(* Logix 5000 AddOnInstructionDefinition export AMCI_MA_SV_Circular_Follower; software revision 31.02 *)

TYPE AMCI_Motion_Axis_Input_Data :
STRUCT
   Moving_CW : BOOL;
   Moving_CCW : BOOL;
   In_Hold_State : BOOL;
   Stopped : BOOL;
   At_Home : BOOL;
   Accelerating : BOOL;
   Decelerating : BOOL;
   Move_Complete : BOOL;
   Status_Word_0_Bit_8 : BOOL;
   Status_Word_0_Bit_9 : BOOL;
   Position_Invalid : BOOL;
   Input_Error : BOOL;
   Command_Error : BOOL;
   Configuration_Error : BOOL;
   Module_OK : BOOL;
   Mode_Flag : BOOL;
   IN1_Active : BOOL;
   IN2_Active : BOOL;
   IN3_Active : BOOL;
   IN4_Active : BOOL;
   Status_Word_1_Bit_4 : BOOL;
   Status_Word_1_Bit_5 : BOOL;
   Connection_Was_Lost : BOOL;
   Driver_Fault : BOOL;
   Status_Word_1_Bit_8 : BOOL;
   Invalid_Jog_Change : BOOL;
   Status_Word_1_Bit_10 : BOOL;
   Heartbeat_Bit : BOOL;
   Status_Word_1_Bit_12 : BOOL;
   Status_Word_1_Bit_13 : BOOL;
   Stall_Detected : BOOL;
   Drive_Is_Enabled : BOOL;
   Motor_Position : DINT;
   Encoder_Position : DINT;
   Trapped_Encoder_Position : DINT;
   Input_Word_8 : INT;
   Input_Word_9 : INT;
END_STRUCT
END_TYPE

TYPE AMCI_Motion_Axis_Output_Data :
STRUCT
   Control_Word_0 : INT;
   Control_Word_1 : INT;
   Position_or_Distance : DINT;
   Programmed_Speed : DINT;
   Acceleration : INT;
   Deceleration : INT;
   Output_Word_8 : INT;
   Output_Word_9 : INT;
END_STRUCT
END_TYPE

ADD_ON_INSTRUCTION AMCI_MA_SV_Circular_Follower   (* revision 1.1, vendor AMCI, ExecuteEnableInFalse *)
// Only for SVXXXE2 motion devices.
// Revision note:
// Version 1.1:  Corrected mistake in the text on the Help Tab.   Also limited the velocity to +/-1,048,575 steps / sec.
// Help:
// MOTION AXIS SV CIRCULAR FOLLOWER
// These AOIs will only work with the SV motion devices.  The SMD and SD  motion devices have their own follower AOIs.
// AXIS INPUT DATA:  Input data from AMCI motion device.   Uses the AMCI_Motion_Axis_Input_Data User Defined Data Type.
// AXIS OUTPUT DATA; Output data from the AOI to the AMCI motion device.   Uses the AMCI_Motion_Axis_Output_Data User Defined Data Type.
// FOLLOWER POSITION: REAL DATA TYPE position directly from the motion axis.
// FOLLOWER VELOCITY: REAL DATA TYPE velocity directly from the motion axis.
// FOLLOWER ACCELERATION: REAL DATA TYPE acceleration directly from the motion axis.
// RAMP ACCELERATION: An actual value or INT value used to transition from no motion to motion.   Once
//                                          motion is occurring, the follower acceleration will be used.  Range of 0 to 15,999.
// DECELERATION: An actual value or INT value used to transition from motion to no motion.   Range of 0 to
//                              15,999.
// CONVERSION CONSTANT: Converts revolutions and revolutions / sec  from the motion axis to the step and
//                                               steps / sec used by the motion axis.
// POSITION UNWIND: Must be set to the Unwind Value of the motion axis and defines the point at which the
//                                    position data will transition from its maximum to its minimum value.    The Position
//                                    Unwind Value MUST BE IN THE RANGE OF 21 TO 65535.
// EN (Enable) Set when rung is true, Reset when rung is false
// DN (Done) Set when command is sent to the motion device.  Reset when the rung is false.
// ER (Error) Set when a command or input error failed to clear.  Reset when the rung is false.
// IP (In Process) Set when motion is occurring.   Reset when the rung goes false.
VAR_IN_OUT
   Axis_Input_Data : AMCI_Motion_Axis_Input_Data; {required}
   Axis_Output_Data : AMCI_Motion_Axis_Output_Data; {required}
END_VAR
VAR_INPUT
   Follower_Position : REAL; {required}
   Follower_Velocity : REAL; {required}
   Follower_Acceleration : REAL; {required}
   Ramp_Acceleration : INT; {required}
   Deceleration : INT; {required}
   Conversion_Constant : REAL; {required}
   Position_Unwind : DINT; {required}
   Maximum_Move_Torque : INT;
END_VAR
VAR_OUTPUT
   EN : BOOL; {visible}
   ER : BOOL; {visible}
   DN : BOOL; {access Read Only, visible}
   IP : BOOL; {access Read Only, visible}
END_VAR
VAR
   command_data_block : INT[10];
        [0]   // Command Bits MSW
        [1]   // Command Bits LSW
        [2]   // Upper Target Position
        [3]   // Lower Target Position
        [4]   // Upper Programmed Speed
        [5]   // Lower Programmed Speed
        [8]   // Unwind value when stopped, Maximum Move Torque when motion occurring
   axis_follower_position : DINT;
   axis_follower_velocity : DINT;
   axis_follower_acceleration : DINT; {access None}
END_VAR

ROUTINE EnableInFalse   (* ladder *)
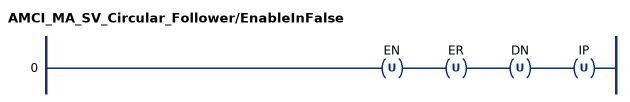
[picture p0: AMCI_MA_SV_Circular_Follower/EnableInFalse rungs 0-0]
   0: OTU(EN)OTU(ER)OTU(DN)OTU(IP);
END_ROUTINE

ROUTINE Logic   (* ladder *)
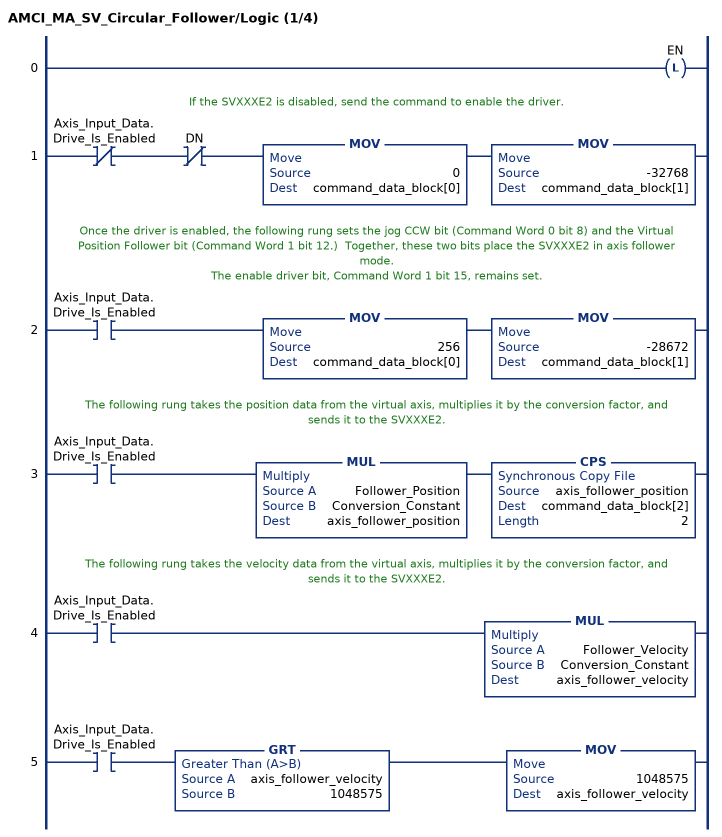
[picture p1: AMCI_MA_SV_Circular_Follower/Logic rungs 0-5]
   0: OTL(EN);
   // If the SVXXXE2 is disabled, send the command to enable the driver.
   1: XIO(Axis_Input_Data.Drive_Is_Enabled)XIO(DN)MOV(0,command_data_block[0])MOV(-32768,command_data_block[1]);
   // Once the driver is enabled, the following rung sets the jog CCW bit (Command Word 0 bit 8) and the Virtual Position Follower bit (Command Word 1 bit 12.)  Together, these two bits place the SVXXXE2 in axis follower mode.
   // The enable driver bit, Command Word 1 bit 15, remains set.
   2: XIC(Axis_Input_Data.Drive_Is_Enabled)MOV(256,command_data_block[0])MOV(-28672,command_data_block[1]);
   // The following rung takes the position data from the virtual axis, multiplies it by the conversion factor, and sends it to the SVXXXE2.
   3: XIC(Axis_Input_Data.Drive_Is_Enabled)MUL(Follower_Position,Conversion_Constant,axis_follower_position)CPS(axis_follower_position,command_data_block[2],2);
   // The following rung takes the velocity data from the virtual axis, multiplies it by the conversion factor, and sends it to the SVXXXE2.
   4: XIC(Axis_Input_Data.Drive_Is_Enabled)MUL(Follower_Velocity,Conversion_Constant,axis_follower_velocity);
   5: XIC(Axis_Input_Data.Drive_Is_Enabled)GRT(axis_follower_velocity,1048575)MOV(1048575,axis_follower_velocity);
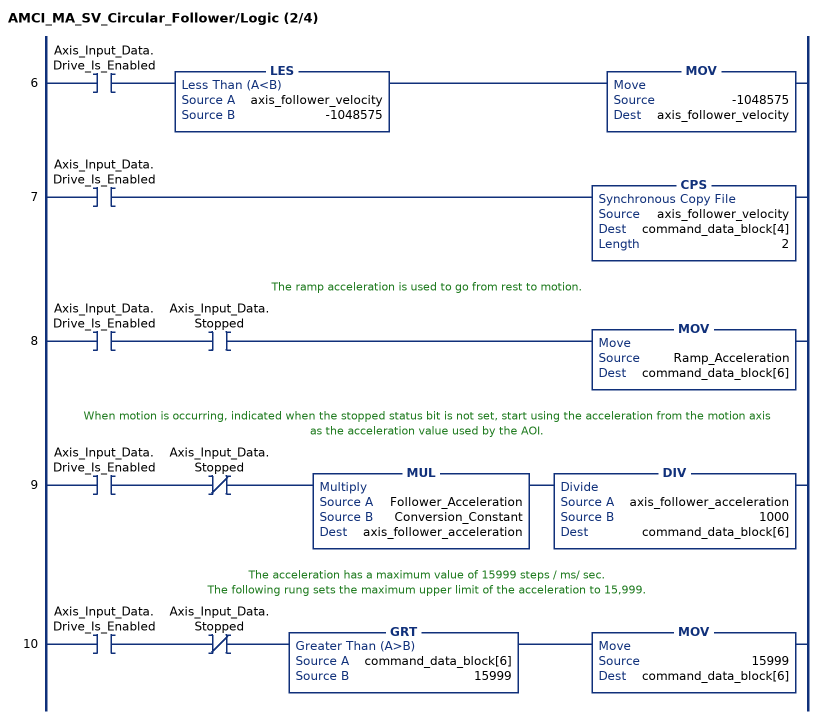
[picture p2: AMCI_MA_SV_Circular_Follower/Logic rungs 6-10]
   6: XIC(Axis_Input_Data.Drive_Is_Enabled)LES(axis_follower_velocity,-1048575)MOV(-1048575,axis_follower_velocity);
   7: XIC(Axis_Input_Data.Drive_Is_Enabled)CPS(axis_follower_velocity,command_data_block[4],2);
   // The ramp acceleration is used to go from rest to motion.
   8: XIC(Axis_Input_Data.Drive_Is_Enabled)XIC(Axis_Input_Data.Stopped)MOV(Ramp_Acceleration,command_data_block[6]);
   // When motion is occurring, indicated when the stopped status bit is not set, start using the acceleration from the motion axis as the acceleration value used by the AOI.
   9: XIC(Axis_Input_Data.Drive_Is_Enabled)XIO(Axis_Input_Data.Stopped)MUL(Follower_Acceleration,Conversion_Constant,axis_follower_acceleration)DIV(axis_follower_acceleration,1000,command_data_block[6]);
   // The acceleration has a maximum value of 15999 steps / ms/ sec.
   // The following rung sets the maximum upper limit of the acceleration to 15,999.
   10: XIC(Axis_Input_Data.Drive_Is_Enabled)XIO(Axis_Input_Data.Stopped)GRT(command_data_block[6],15999)MOV(15999,command_data_block[6]);
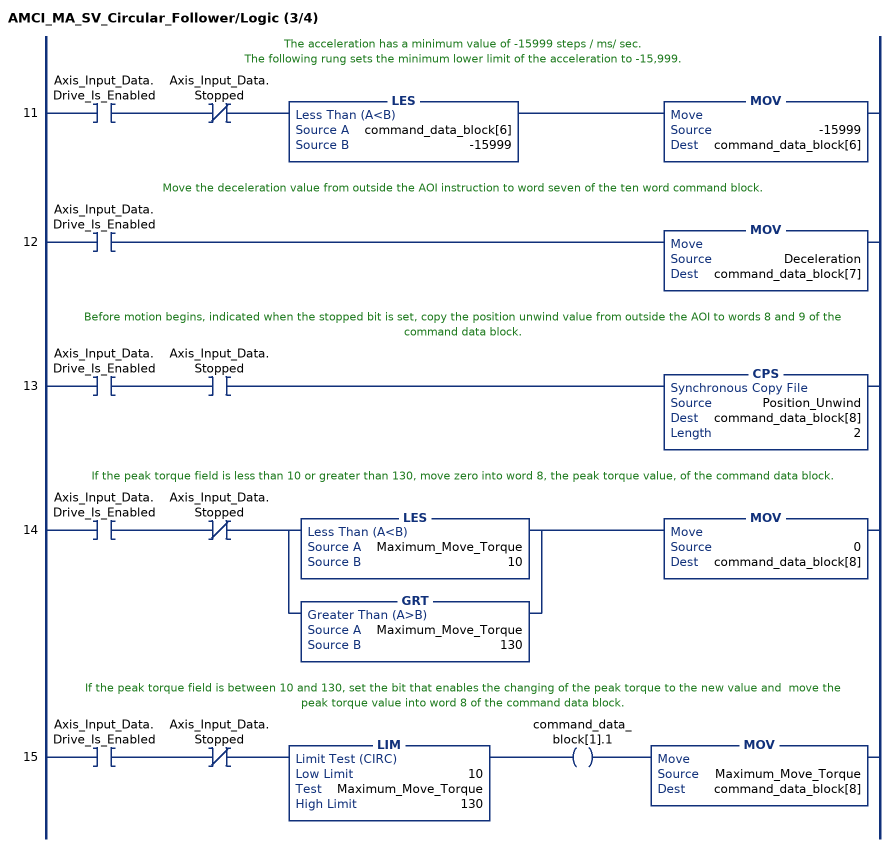
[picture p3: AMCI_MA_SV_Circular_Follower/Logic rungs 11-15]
   // The acceleration has a minimum value of -15999 steps / ms/ sec.
   // The following rung sets the minimum lower limit of the acceleration to -15,999.
   11: XIC(Axis_Input_Data.Drive_Is_Enabled)XIO(Axis_Input_Data.Stopped)LES(command_data_block[6],-15999)MOV(-15999,command_data_block[6]);
   // Move the deceleration value from outside the AOI instruction to word seven of the ten word command block.
   12: XIC(Axis_Input_Data.Drive_Is_Enabled)MOV(Deceleration,command_data_block[7]);
   // Before motion begins, indicated when the stopped bit is set, copy the position unwind value from outside the AOI to words 8 and 9 of the command data block.
   13: XIC(Axis_Input_Data.Drive_Is_Enabled)XIC(Axis_Input_Data.Stopped)CPS(Position_Unwind,command_data_block[8],2);
   // If the peak torque field is less than 10 or greater than 130, move zero into word 8, the peak torque value, of the command data block.
   14: XIC(Axis_Input_Data.Drive_Is_Enabled)XIO(Axis_Input_Data.Stopped)[LES(Maximum_Move_Torque,10) ,GRT(Maximum_Move_Torque,130) ]MOV(0,command_data_block[8]);
   // If the peak torque field is between 10 and 130, set the bit that enables the changing of the peak torque to the new value and  move the peak torque value into word 8 of the command data block.
   15: XIC(Axis_Input_Data.Drive_Is_Enabled)XIO(Axis_Input_Data.Stopped)LIM(10,Maximum_Move_Torque,130)OTE(command_data_block[1].1)MOV(Maximum_Move_Torque,command_data_block[8]);
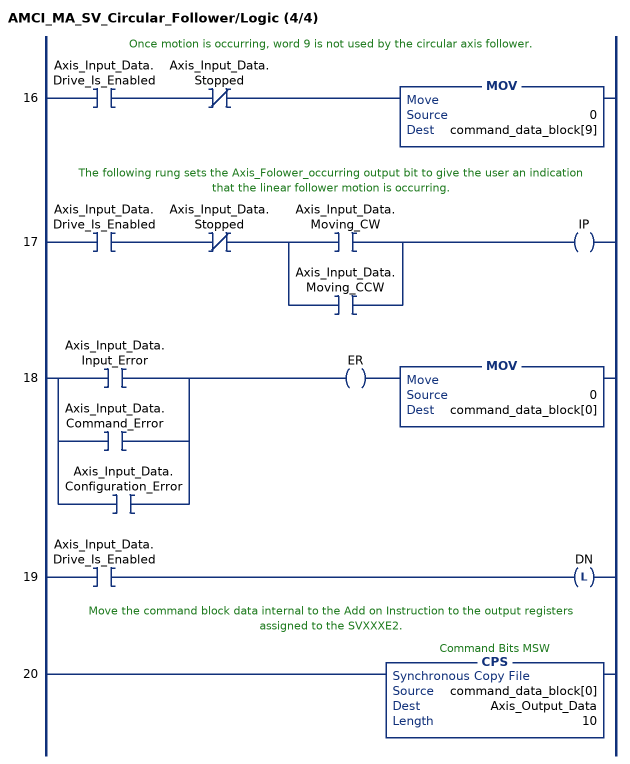
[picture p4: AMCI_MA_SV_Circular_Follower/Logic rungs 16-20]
   // Once motion is occurring, word 9 is not used by the circular axis follower.
   16: XIC(Axis_Input_Data.Drive_Is_Enabled)XIO(Axis_Input_Data.Stopped)MOV(0,command_data_block[9]);
   // The following rung sets the Axis_Folower_occurring output bit to give the user an indication that the linear follower motion is occurring.
   17: XIC(Axis_Input_Data.Drive_Is_Enabled)XIO(Axis_Input_Data.Stopped)[XIC(Axis_Input_Data.Moving_CW) ,XIC(Axis_Input_Data.Moving_CCW) ]OTE(IP);
   18: [XIC(Axis_Input_Data.Input_Error) ,XIC(Axis_Input_Data.Command_Error) ,XIC(Axis_Input_Data.Configuration_Error) ]OTE(ER)MOV(0,command_data_block[0]);
   19: XIC(Axis_Input_Data.Drive_Is_Enabled)OTL(DN);
   // Move the command block data internal to the Add on Instruction to the output registers assigned to the SVXXXE2.
   20: CPS(command_data_block[0],Axis_Output_Data,10);
END_ROUTINE
END_ADD_ON_INSTRUCTION
